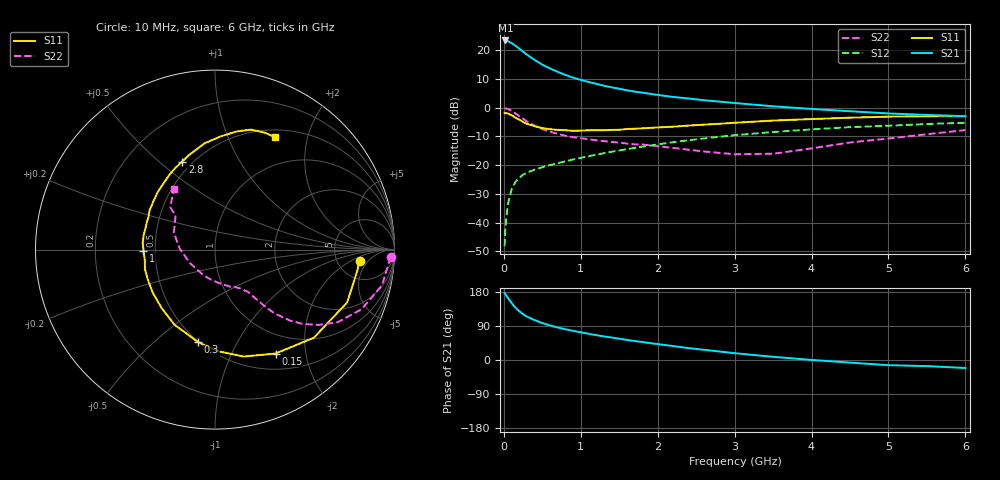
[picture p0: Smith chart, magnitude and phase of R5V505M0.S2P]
! SIEMENS Small Signal Semiconductors
! BFR183
! Si NPN RF Bipolar Junction Transistor in SOT23
! VCE = 0.5 V  IC = 5 mA
! Common Emitter S-Parameters:  May  1996
# GHz  S  MA  R  50
!  f  S11  S21  S12  S22
! GHz  MAG  ANG  MAG  ANG  MAG  ANG  MAG  ANG
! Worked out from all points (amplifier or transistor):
!   36 points, 10 MHz to 6 GHz, reference 50 ohm
!   highest |S21| = 23.4 dB at 20 MHz (marker M1)
!   |S21| within 3 dB of that: start of sweep to 207.4 MHz
!   unconditionally stable (mu >= 1): 888.7 MHz to 3.484 GHz
!   at 250 MHz: K = 0.44, MSG = 21.4 dB, |S12| = -23.3 dB
!   at 1.4 GHz: K = 1.10, MAG = 9.2 dB, |S12| = -15.4 dB
!   at 6 GHz: K = 0.98, MSG = 1.1 dB, |S12| = -5.3 dB
!   S11 on the Smith chart (normalised r, x): 10 MHz: 8.30, -3.03; 150 MHz: 0.71, -1.49; 300 MHz: 0.50, -0.71; 1 GHz: 0.43, -0.01; 2.8 GHz: 0.44, +0.60; 6 GHz: 0.59, +1.50
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0.01  0.808 -4.5  14.61 177.2  0.0039 86.2  0.9789 -2.4
0.02  0.8011 -8.7  14.73 173.6  0.0082 84.7  0.9695 -4.8
0.05  0.793 -21.8  14.38 164.7  0.0202 78.2  0.9517 -12.0
0.1  0.738 -41.7  13.29 150.9  0.0375 69.9  0.882 -22.1
0.15  0.6701 -59.8  12 138.2  0.0508 61.6  0.7946 -30.6
0.2  0.6172 -74.9  10.62 129.0  0.0607 56.9  0.7127 -36.1
0.25  0.5659 -88.5  9.381 121.0  0.0683 53.3  0.6401 -40.3
0.3  0.524 -100.3  8.361 114.5  0.0739 51.3  0.5762 -43.4
0.4  0.4755 -118.4  6.758 105.3  0.0837 48.8  0.4849 -47.0
0.5  0.4408 -132.5  5.579 97.6  0.092 48.3  0.4246 -48.6
0.6  0.4216 -145.4  4.803 91.2  0.1002 48.5  0.3819 -49.6
0.8  0.4051 -164.3  3.71 81.1  0.1164 49.4  0.3243 -51.1
1  0.3984 -179.2  3.038 73.1  0.1336 50.1  0.2947 -52.5
1.1  0.4043 175.0  2.798 69.3  0.1427 50.5  0.2826 -53.9
1.3  0.4049 163.7  2.411 62.3  0.1612 50.5  0.2617 -56.2
1.6  0.4249 149.1  1.999 52.9  0.1897 50.0  0.2368 -61.6
2.2  0.4667 128.1  1.535 36.7  0.2505 46.3  0.1997 -77.1
2.8  0.5236 110.4  1.275 22.5  0.3113 40.3  0.1634 -103.5
3.5  0.5955 95.5  1.055 8.4  0.3766 31.3  0.1578 -151.1
4.5  0.6686 79.7  0.866 -6.9  0.4582 18.6  0.2477 157.7
5.5  0.7078 67.0  0.746 -16.1  0.5191 7.0  0.3444 136.5
6  0.7111 61.8  0.71 -21.1  0.5453 -0.5  0.4076 123.8
